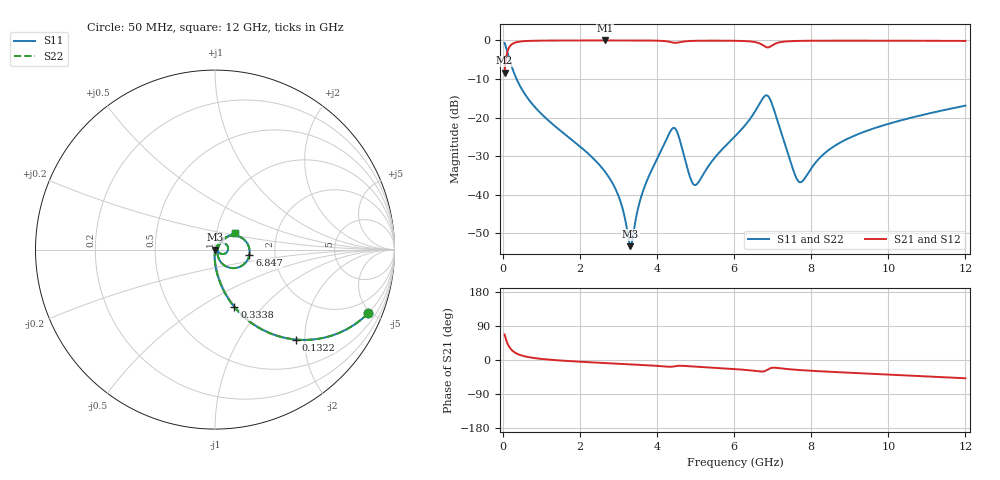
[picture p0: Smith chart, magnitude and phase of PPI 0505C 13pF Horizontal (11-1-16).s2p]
# MHz S MA R 50
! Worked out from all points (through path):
!   1601 points, 50 MHz to 12 GHz, reference 50 ohm
!   highest |S21| = -0.02 dB at 2.657 GHz (marker M1); lowest = -8.4 dB at 50 MHz (marker M2)
!   group delay of S21, straight-line fit = 13.3 ps
!   lowest |S11| = -53.4 dB at 3.314 GHz (marker M3), VSWR 1.00, Z = 50.2 - j0.0643 ohm
!   |S11| at or under -10 dB: 359.8 MHz to end of sweep
!   |S22| runs from -53.4 to -0.7 dB; largest |S21 - S12| = 0
!   S11 on the Smith chart (normalised r, x): 50 MHz: 0.99, -4.81; 132.2 MHz: 0.99, -1.82; 333.8 MHz: 0.99, -0.71; 6.847 GHz: 1.47, -0.09; 12 GHz: 1.22, +0.23
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50  0.9243 -22.6  0.3817 67.4  0.3817 67.4  0.9243 -22.6
132.1562  0.675 -48.0  0.7375 42.0  0.7375 42.0  0.675 -48.0
333.8125  0.3385 -71.3  0.9404 18.6  0.9404 18.6  0.3385 -71.3
886.5  0.1279 -85.4  0.9909 4.3  0.9909 4.3  0.1279 -85.4
2044.156  0.04055 -93.0  0.9978 -4.8  0.9978 -4.8  0.04055 -93.0
2656.594  0.01974 -93.8  0.9981 -8.1  0.9981 -8.1  0.01974 -93.8
3022.562  0.009056 -88.8  0.998 -10.0  0.998 -10.0  0.009056 -88.8
3313.844  0.002145 -17.4  0.9977 -11.5  0.9977 -11.5  0.002145 -17.4
3620.062  0.01041 59.9  0.9967 -13.1  0.9967 -13.1  0.01041 59.9
4038.312  0.03132 58.1  0.9905 -15.7  0.9905 -15.7  0.03132 58.1
4464.031  0.07262 0.2  0.93 -16.7  0.93 -16.7  0.07262 0.2
4867.344  0.0164 -22.0  0.9834 -16.7  0.9834 -16.7  0.0164 -22.0
5001.781  0.01334 10.5  0.9879 -17.6  0.9879 -17.6  0.01334 10.5
6025  0.05707 56.0  0.9881 -24.0  0.9881 -24.0  0.05707 56.0
6629.969  0.1416 32.9  0.9271 -30.0  0.9271 -30.0  0.1416 32.9
6846.562  0.1938 -9.0  0.8133 -26.9  0.8133 -26.9  0.1938 -9.0
7152.781  0.08264 -63.9  0.9371 -21.3  0.9371 -21.3  0.08264 -63.9
7638.25  0.01564 -29.5  0.9839 -26.1  0.9839 -26.1  0.01564 -29.5
8019.156  0.02253 35.8  0.9895 -28.5  0.9895 -28.5  0.02253 35.8
8728.688  0.04655 49.7  0.9919 -32.3  0.9919 -32.3  0.04655 49.7
10013.31  0.083 47.9  0.9908 -38.6  0.9908 -38.6  0.083 47.9
12000  0.1424 39.7  0.984 -48.2  0.984 -48.2  0.1424 39.7
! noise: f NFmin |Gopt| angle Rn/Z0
50  0.0003871  0.8676  1.62  0.0006286
1372  0.003802  0.6612  5.16  0.002142
2701  0.006524  0.6216  9.512  0.003198
4031  0.0185  0.7823  13.91  0.01718
5360  0.02025  0.7432  18.43  0.01543
6682  0.07826  0.91  22.9  0.1838
8012  0.0278  0.7281  27.28  0.01924
9341  0.02278  0.6379  31.28  0.01104
1.067e+04  0.02312  0.6058  35.14  0.009913
1.2e+04  0.02458  0.5927  38.89  0.009918
